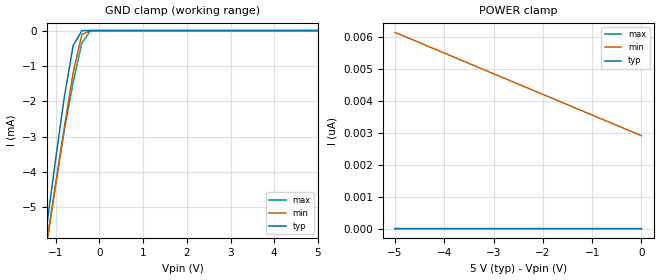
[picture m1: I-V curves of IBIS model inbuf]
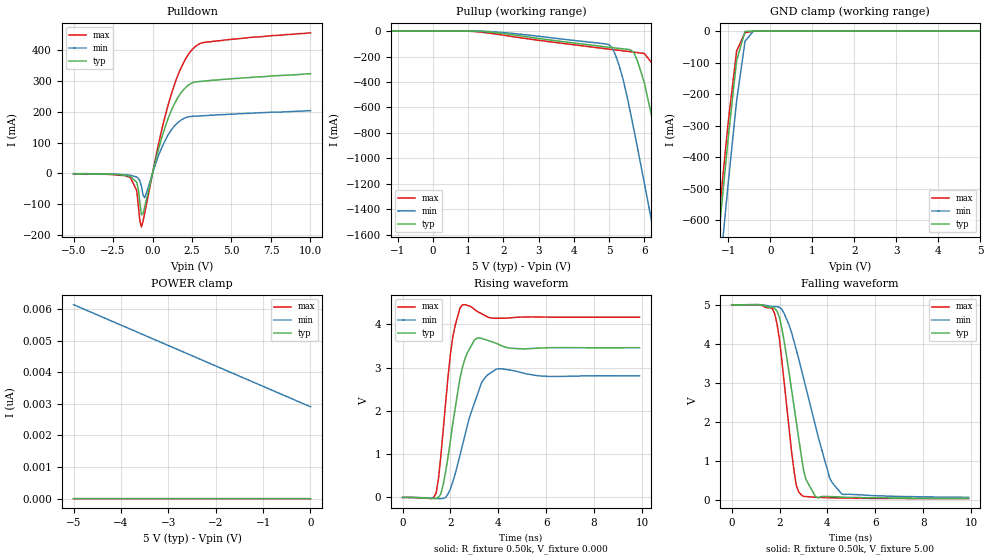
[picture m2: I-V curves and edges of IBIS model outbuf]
| IBIS file 41823h.ibs created by s2ibis2 version 1.0
| North Carolina State University Electronics Research Laboratory  1995
[IBIS ver]   2.1
[File name]   41823h.ibs
[File Rev]   0.1
[Date]   Thursday, May 17, 2001
[Source]   IDT
[Notes]   1. Temp typ=25C, min=100C, max=0C 2. Ramp rates based on 500
   ohm load
[Copyright]   Copyright 2001, Integrated Device Technology, Inc.
[Disclaimer] Integrated Device Technology, Inc. ("IDT") hereby grants the
   user of this IBIS model a non-exclusive, nontransferable
   license to use this IBIS model under the following terms.
   The user is granted this license only to use the IBIS model
   and is not granted rights to sell, copy (except as needed to
   run the IBIS model), rent, lease or sub-license the IBIS model
   in whole or in part, or in modified form to anyone.
   The User may modify the IBIS model to suit its specific
   applications, but rights to derivative works and such
   modifications shall belong to IDT.
   This IBIS model is provided on an "AS IS" basis and IDT
   makes absolutely no warranty with respect to the information
   contained herein. IDT DISCLAIMS AND CUSTOMER WAIVES ALL
   WARRANTIES, EXPRESS AND IMPLIED, INCLUDING WARRANTIES OF
   MERCHANTABILITY AND FITNESS FOR A PARTICULAR PURPOSE. THE
   ENTIRE RISK AS TO QUALITY AND PERFORMANCE IS WITH THE
   USER ACCORDINGLY, IN NO EVENT SHALL IDT BE LIABLE
   FOR ANY DIRECT OR INDIRECT DAMAGES, WHETHER IN CONTRACT OR
   TORT, INCLUDING ANY LOST PROFITS OR OTHER INCIDENTAL,
   CONSEQUENTIAL, EXEMPLARY, OR PUNITIVE DAMAGES ARISING OUT OF
   THE USE OR APPLICATION OF THE IBIS model.  Further, IDT
   reserves the right to make changes without notice to any
   product herein to improve reliability, function, or design.
   IDT does not convey any license under patent rights or
   any other intellectual property rights, including those of
   third parties. IDT is not obligated to provide maintenance
   or support for the licensed IBIS model.
|   Component IDT54/74FCT823T/AT/CT
[Component]   IDT54/74FCT823T/AT/CT
[Manufacturer]   Integrated Device Technology Inc.
[Package]
| Following package parameters are for D20-1(CDIP), P20-1(DPIP) packages
|[Package]
|| variable   typ   min   max
|R_pkg   40.00m   30.00m   50.00m
|L_pkg   7.00nH   4.00nH   10.00nH
|C_pkg   0.60pF   0.50pF   0.70pF
| Following package parameters are for SO20-6(EIAJ), SO20-2(SOIC) packages
|[Package]
|| variable   typ   min   max
|R_pkg   25.00m   20.00m   30.00m
|L_pkg   3.50nH   2.10nH   6.50nH
|C_pkg   0.40pF   0.35pF   0.60pF
| Following package parameters are for SO20-8(QSOP), SO20-7(SSOP) packages
| variable   typ   min   max
R_pkg   20.00m   15.00m   25.00m
L_pkg   3.00nH   2.00nH   4.00nH
C_pkg   0.30pF   0.26pF   0.34pF
[Pin]  signal_name   model_name   R_pin   L_pin   C_pin
1   OEB   inbuf
2   D0   inbuf
3   D1   inbuf
4   D2   inbuf
5   D3   inbuf
6   D4   inbuf
7   D5   inbuf
8   D6   inbuf
9   D7   inbuf
10   D8   inbuf
11   CLRB   inbuf
12   GND   GND
13   CP   inbuf
14   ENB   inbuf
15   Y8   outbuf
16   Y7   outbuf
17   Y6   outbuf
18   Y5   outbuf
19   Y4   outbuf
20   Y3   outbuf
21   Y2   outbuf
22   Y1   outbuf
23   Y0   outbuf
24   VCC   POWER
| Models and submodels in the file (2): inbuf (Input), outbuf (3-state)
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| in   IN1   dummy_model
| oe   OE1   dummy_model
|   Model inbuf
[Model]   inbuf
Model_type   Input
Vinl =  0.800V
Vinh =  2.000V
C_comp   3.00pF   NA   NA
[Temperature Range]   25.00   100.00   0.000
[Voltage Range]   5.00V   4.50V   5.50V
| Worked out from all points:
|   GND clamp passes 1 mA (typ) near -0.68 V on its own axis
[GND_clamp]
| voltage   I(typ)   I(min)   I(max)
-5V       -42.6mA    -38.92mA   -44.14mA
-1.4V     -7.395mA   -7.704mA   -7.764mA
-1.2V     -5.498mA   -6.015mA   -5.991mA
-1V       -3.639mA   -4.348mA   -4.354mA
-800mV    -1.867mA   -2.722mA   -2.8mA
-600mV    -428uA     -1.196mA   -1.467mA
-400mV    -308nA     -110uA     -354uA
-200mV    -128pA     -324nA     -3.818pA
5V        467fA      3.232nA    200fA
[POWER_clamp]
| voltage   I(typ)   I(min)   I(max)
-5V       995fA      6.14nA     492fA
-1.1V     584fA      3.62nA     285fA
-300mV    499fA      3.102nA    242fA
0V        467fA      2.909nA    226fA
|   Model outbuf
[Model]   outbuf
Model_type   3-state
Polarity   Non-Inverting
Enable   Active-High
Vinl =  0.800V
Vinh =  2.000V
C_comp   3.00pF   NA   NA
[Temperature Range]   25.00   100.00   0.000
[Voltage Range]   5.00V   4.50V   5.50V
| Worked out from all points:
|   slope of the pulldown table from 0 to 0.75 V, typ, clamps not added: 5.24 ohm
|   GND clamp passes 1 mA (typ) near -0.55 V on its own axis
|   rising waveform, R_fixture 0.50k, V_fixture 0.000: 20-80 % time 575ps typ, 839ps min, 430ps max; typ from 0 V to 3.46 V
|   falling waveform, R_fixture 0.50k, V_fixture 5.00: 20-80 % time 728ps typ, 1.25ns min, 530ps max; typ from 5 V to 0.048 V
[Pulldown]
| voltage   I(typ)   I(min)   I(max)
-5V       -1mA       -1mA       -2mA
-1.4V     -9.8mA     -6mA       -13.4mA
-1V       -29mA      -12.1mA    -56.2mA
-800mV    -96.14mA   -24.2mA    -155mA
-700mV    -135mA     -41.6mA    -174mA
-500mV    -110mA     -79.11mA   -130mA
300mV     63.4mA     46.63mA    75.9mA
900mV     166mA      117mA      206mA
1.7V      254mA      169mA      331mA
2.5V      294mA      185mA      402mA
3.4V      301mA      188mA      427mA
10V       324mA      204mA      457mA
[Pullup]
| voltage   I(typ)   I(min)   I(max)
-5V       0A         0A         0A
1V        -8.847nA   2.262nA    -1.229mA
5V        -127mA     -107mA     -142mA
5.2V      -134mA     -202mA     -149mA
5.4V      -140mA     -383mA     -156mA
5.7V      -168mA     -770mA     -166mA
6V        -407mA     -1.193A    -176mA
6.4V      -907mA     -1.772A    -316mA
6.8V      -1.479A    -2.358A    -720mA
7.2V      -2.062A    -2.947A    -1.276A
7.6V      -2.649A    -3.538A    -1.851A
10V       -6.198A    -7.105A    -5.355A
[GND_clamp]
| voltage   I(typ)   I(min)   I(max)
-5V       -6.197A    -6.359A    -6.087A
-1.4V     -897mA     -1.044A    -841mA
-1.2V     -613mA     -759mA     -560mA
-1V       -338mA     -482mA     -289mA
-800mV    -93.56mA   -221mA     -62.93mA
-600mV    -1.295mA   -32.12mA   -4.927mA
-400mV    -309nA     -162uA     -676uA
5V        468fA      3.232nA    198fA
[POWER_clamp]
| voltage   I(typ)   I(min)   I(max)
-5V       995fA      6.14nA     489fA
-1.1V     584fA      3.62nA     286fA
-300mV    502fA      3.102nA    244fA
0V        467fA      2.909nA    227fA
[Ramp]
| variable   typ   min   max
dV/dt_r   2.07/0.58n   1.68/0.84n   2.50/0.43n
dV/dt_f   2.97/0.73n   2.66/1.16n   3.27/0.57n
R_load = 0.50k
[Rising Waveform]
R_fixture = 0.50k
V_fixture = 0.000
| time   V(typ)   V(min)   V(max)
0s        0V         0V         0V
1.4ns     -21.38mV   -24.12mV   101mV
1.5ns     4.617mV    -28.29mV   435mV
1.7ns     306mV      -21.1mV    1.576V
2.1ns     1.719V     364mV      3.715V
2.5ns     3.004V     1.203V     4.449V
3ns       3.634V     2.177V     4.344V
3.3ns     3.673V     2.651V     4.243V
3.9ns     3.56V      2.959V     4.137V
9.9ns     3.457V     2.808V     4.163V
[Falling Waveform]
R_fixture = 0.50k
V_fixture = 5.00
| time   V(typ)   V(min)   V(max)
0s        5V         5V         5V
1.8ns     4.905V     4.955V     4.766V
2.1ns     4.386V     4.877V     3.553V
2.6ns     2.423V     4.073V     775mV
2.9ns     1.18V      3.374V     143mV
3.1ns     536mV      2.888V     93.34mV
3.5ns     96.21mV    1.908V     76.58mV
4.1ns     92.8mV     561mV      62.66mV
4.6ns     80.03mV    159mV      56.01mV
9.9ns     48.12mV    74.23mV    39.36mV
